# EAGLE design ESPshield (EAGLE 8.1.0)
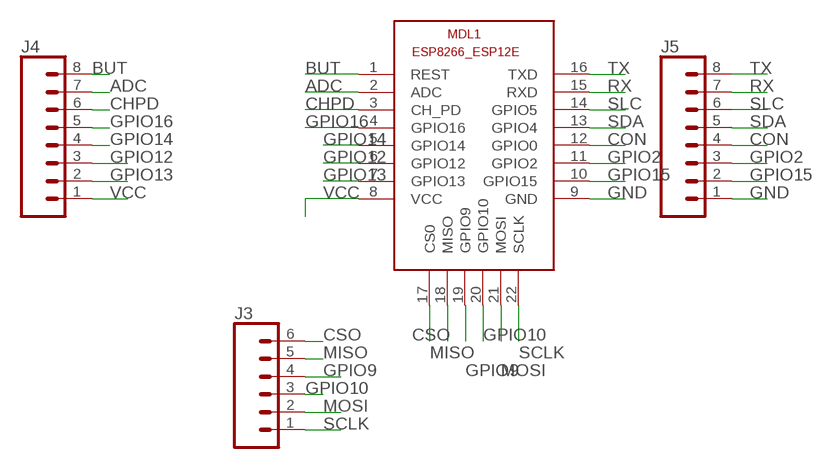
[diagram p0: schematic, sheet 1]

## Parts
J3  CONN_06LONGPADS  [1X06_LONGPADS]
J4  CONN_08LONGPADS  [1X08_LONGPADS]
J5  CONN_08LONGPADS  [1X08_LONGPADS]
MDL1  ESP8266-12EESP8266-ESP12E  [ESP8266-ESP12E]

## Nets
ADC: J4.7 MDL1.2(ADC)
BUT: J4.8 MDL1.1(REST)
CHPD: J4.6 MDL1.3(CH_PD)
CON: J5.4 MDL1.12(GPIO0)
CSO: J3.6 MDL1.17(CS0)
GND: J5.1 MDL1.9(GND)
GPIO2: J5.3 MDL1.11(GPIO2)
GPIO9: J3.4 MDL1.19(GPIO9)
GPIO10: J3.3 MDL1.20(GPIO10)
GPIO12: J4.3 MDL1.6(GPIO12)
GPIO13: J4.2 MDL1.7(GPIO13)
GPIO14: J4.4 MDL1.5(GPIO14)
GPIO15: J5.2 MDL1.10(GPIO15)
GPIO16: J4.5 MDL1.4(GPIO16)
MISO: J3.5 MDL1.18(MISO)
MOSI: J3.2 MDL1.21(MOSI)
RX: J5.7 MDL1.15(RXD)
SCLK: J3.1 MDL1.22(SCLK)
SDA: J5.5 MDL1.13(GPIO4)
SLC: J5.6 MDL1.14(GPIO5)
TX: J5.8 MDL1.16(TXD)
VCC: J4.1 MDL1.8(VCC)

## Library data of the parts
J3 = SparkFun-Connectors:CONN_06: Multi connection point. Often used as Generic Header-pin footprint for 0.1 inch spaced/style header connections On any of the 0.1 inch spaced packages, you can populate with these: Break Away Headers - Straight (PRT-00116) Break Away Male Headers - Right Angle (PRT-00553) Female Headers (PRT-00115)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
J4 J5 = SparkFun-Connectors:CONN_08: Multi connection point. Often used as Generic Header-pin footprint for 0.1 inch spaced/style header connections On any of the 0.1 inch spaced packages, you can populate with these: Break Away Headers - Straight (PRT-00116) Break Away Male Headers - Right Angle (PRT-00553) Female Headers (PRT-00115)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
MDL1 = ESP8266-ESP12E:ESP8266-12E: ESP8266-12E with additional I/O and GPIO04/05 corrected The author cannot warrant that this library is free from error or will meet your specific requirements. Created by PuceBaboon.com. Komagane, Nagano, JAPAN

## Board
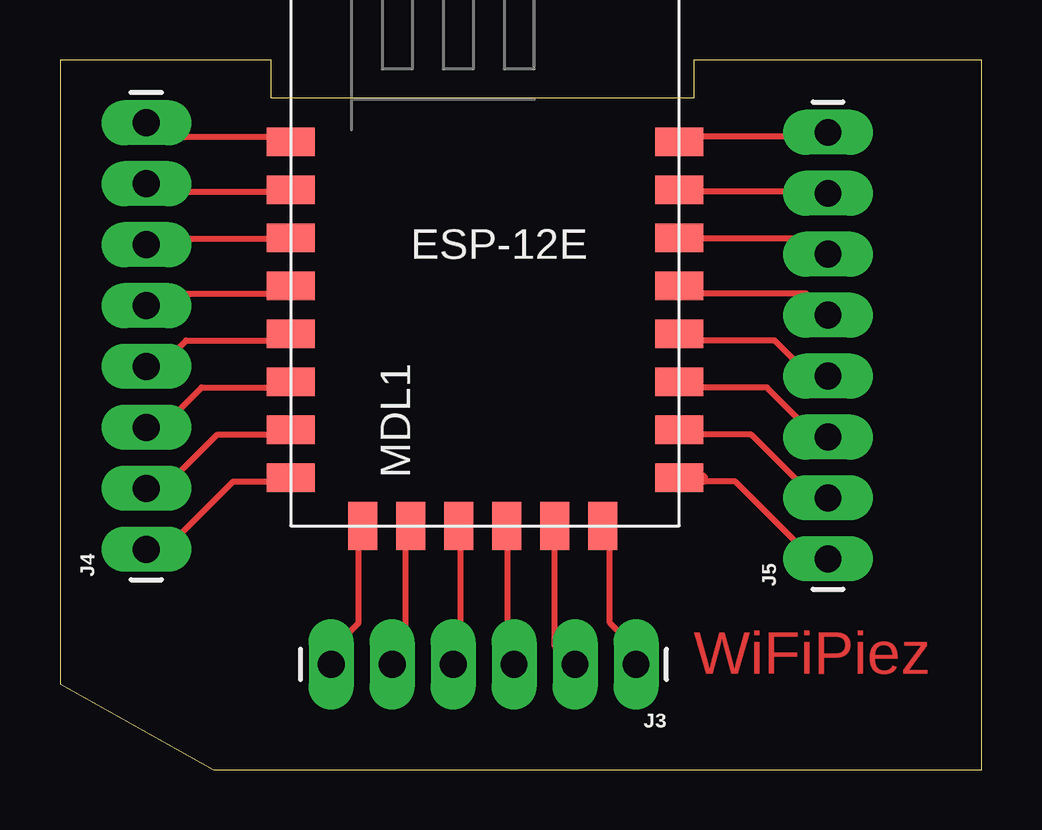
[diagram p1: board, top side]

Size 38.4 x 29.6 mm. Coordinates in mm from the lower left corner, seen from the top.
Outline: 0,29.6 0,3.6 6.4,0 38.4,0 38.4,29.6 26.4,29.6 26.4,28 8.8,28 8.8,29.6 0,29.6
Copper layers (1*16): Top 0.035mm / dielectric 1.5mm / Bottom 0.035mm
Design rules "default *": minimum track width 10mil, minimum drill 24mil, track to track 0.4mm, track to pad 0.4mm, pad to pad 0.4mm, via to via 0.4mm, smd to smd 0.4mm, copper to edge 40mil, drill to drill 8mil, minimum pad ring 10mil, minimum via ring 8mil, stop-mask expansion 4mil, vias tented up to drill 0mil, thermal gap 10mil

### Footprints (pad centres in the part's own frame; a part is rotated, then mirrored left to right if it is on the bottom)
1X06_LONGPADS = drill 1.118 pad 1.88 long: 1 0,0; 2 2.54,0; 3 5.08,0; 4 7.62,0; 5 10.16,0; 6 12.7,0
1X08_LONGPADS = drill 1.118 pad 1.88 long: 1 0,0; 2 2.54,0; 3 5.08,0; 4 7.62,0; 5 10.16,0; 6 12.7,0; 7 15.24,0; 8 17.78,0
ESP8266-ESP12E = smd 2 x 1.2: 1 -7.62,5.84; 2 -7.62,3.84; 3 -7.62,1.84; 4 -7.62,-0.16; 5 -7.62,-2.16; 6 -7.62,-4.16; 7 -7.62,-6.16; 8 -7.62,-8.16; 9 8.58,-8.16; 10 8.58,-6.16; 11 8.58,-4.16; 12 8.58,-2.16; 13 8.58,-0.16; 14 8.58,1.84; 15 8.58,3.84; 16 8.58,5.84 | smd 1.2 x 2: 17 -4.62,-10.16; 18 -2.62,-10.16; 19 -0.62,-10.16; 20 1.38,-10.16; 21 3.38,-10.16; 22 5.38,-10.16

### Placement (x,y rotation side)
J3  24,4.4 180 top
J4  3.6,9.2 90 top
J5  32,8.8 90 top
MDL1  17.23,20.34 0 top

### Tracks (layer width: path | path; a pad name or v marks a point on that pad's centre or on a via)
ADC
  Top 0.254: 9.4,24.4 MDL1.2 9.5,24.12 3.62,24.12 J4.7
BUT
  Top 0.254: MDL1.1 9.5,26.41 3.94,26.41 3.62,26.73 J4.8
CHPD
  Top 0.254: 9.4,21.9 MDL1.3 9.5,22.16 3.62,22.16 J4.6
CON
  Top 0.254: 25.9,18.4 MDL1.12 25.85,17.91 29.78,17.91 31.09,16.6 31.74,16.6 J5.4
CSO
  Top 0.254: MDL1.17 12.45,10.06 12.45,6.13 11.46,5.15 11.46,4.5 J3.6
GND
  Top 0.254: 26.8,12.18 26.83,12.02 28.14,12.02 31.09,9.08 31.74,9.08 J5.1
  Top 0.406: MDL1.9 26.8,12.18
GPIO2
  Top 0.254: MDL1.11 25.85,15.94 29.45,15.94 31.74,13.65 J5.3
GPIO9
  Top 0.254: MDL1.19 16.7,10.06 16.7,4.5 J3.4
GPIO10
  Top 0.254: MDL1.20 18.66,10.06 18.66,4.5 J3.3
GPIO12
  Top 0.254: MDL1.6 9.5,15.94 5.91,15.94 4.27,14.31 3.62,14.31 J4.3
GPIO13
  Top 0.254: MDL1.7 9.5,13.98 6.56,13.98 4.6,12.02 3.62,12.02 J4.2
GPIO14
  Top 0.254: MDL1.5 9.5,17.91 5.25,17.91 4.27,16.92 3.62,16.92 J4.4
GPIO15
  Top 0.254: MDL1.10 25.85,13.98 28.8,13.98 31.74,11.04 J5.2
GPIO16
  Top 0.254: MDL1.4 9.5,19.87 3.94,19.87 3.62,19.54 J4.5
MISO
  Top 0.254: MDL1.18 14.41,10.06 14.41,4.83 14.08,4.5 J3.5
MOSI
  Top 0.254: MDL1.21 20.62,10.06 20.62,5.15 21.27,4.5 J3.2
RX
  Top 0.254: MDL1.15 25.85,24.12 31.74,24.12 J5.7
SCLK
  Top 0.254: MDL1.22 22.91,10.06 22.91,6.13 23.89,5.15 23.89,4.5 J3.1
SDA
  Top 0.254: MDL1.13 25.85,19.87 31.09,19.87 31.74,19.21 J5.5
SLC
  Top 0.254: MDL1.14 25.85,22.16 31.09,22.16 31.74,21.5 J5.6
TX
  Top 0.254: MDL1.16 25.85,26.41 31.74,26.41 J5.8
VCC
  Top 0.254: MDL1.8 9.5,12.02 7.21,12.02 4.6,9.4 3.62,9.4 J4.1
  Top 0.406: 10.38,12.18 MDL1.8 9.43,12

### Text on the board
Top: WiFiPiez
